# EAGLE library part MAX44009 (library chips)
low power ambient light sensor
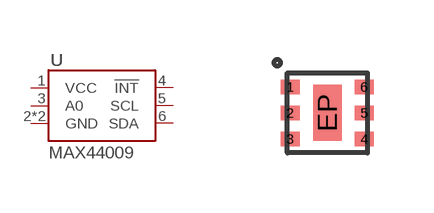
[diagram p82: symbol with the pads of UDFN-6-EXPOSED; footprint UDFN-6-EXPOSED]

Designator prefix U

## MAX44009 (DIGIKEY: MAX44009EDT+TCT-ND; MANUFACTURER: MAXIM; MPN: MAX44009EDT+T)  [UDFN-6-EXPOSED]
1  VCC
2  GND
3  A0
4  !INT
5  SCL
6  SDA
EP  GND

## Footprint UDFN-6-EXPOSED (pad centres in mm)
smd 0.48 x 0.36: 1 -0.925,0.65; 2 -0.925,0; 3 -0.925,-0.65; 4 0.925,-0.65; 5 0.925,0; 6 0.925,0.65
smd 0.71 x 1.4: EP 0,0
